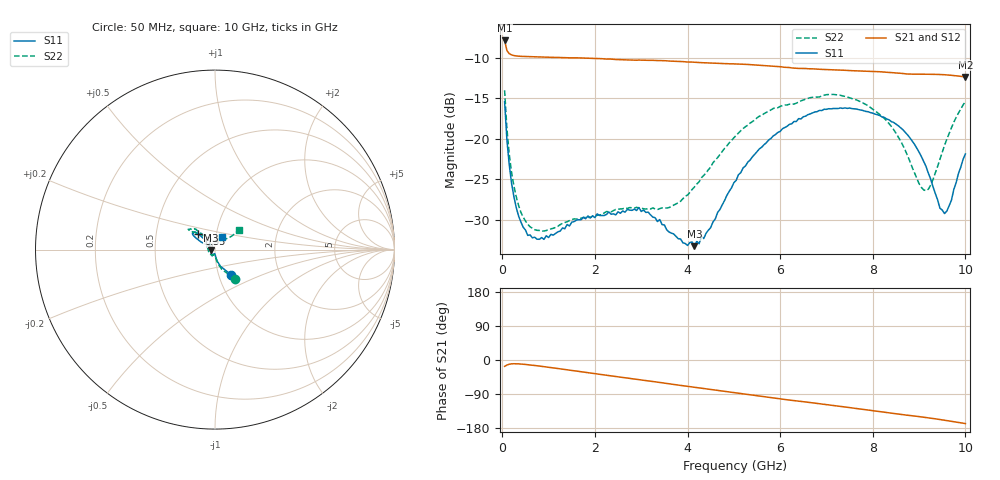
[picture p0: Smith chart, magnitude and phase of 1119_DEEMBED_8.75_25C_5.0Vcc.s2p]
!Hittite Microwave Corp.
!Digital Attenuator/PhaseShifter Rev 1.4.0
!Filename: C:\DATA\DATA\1119_DEEMBED_8.75_25C_5.0Vcc.s2p
!VNA ID: Agilent Technologies,N5224A,MY51441122,A.10.45.03
!Device type:
!2 Port Calibration.
!Temp(C): 25
!Lot Number:
!Serial Number:
!Operator:
!Misc:
!Attenuator:  8.750
# GHZ S DB R 50.0
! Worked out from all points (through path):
!   200 points, 50 MHz to 10 GHz, reference 50 ohm
!   highest |S21| = -7.89 dB at 50 MHz (marker M1); lowest = -12.4 dB at 10 GHz (marker M2)
!   group delay of S21, straight-line fit = 45 ps
!   lowest |S11| = -33.3 dB at 4.15 GHz (marker M3), VSWR 1.04, Z = 47.9 - j0.255 ohm
!   |S11| at or under -10 dB: start of sweep to end of sweep
!   |S22| runs from -31.4 to -14.0 dB; largest |S21 - S12| = 0.00082
!   S11 on the Smith chart (normalised r, x): 50 MHz: 1.15, -0.34; 6.35 GHz: 0.82, +0.15; 10 GHz: 1.07, +0.15
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0.05  -15.45 -57.1  -7.89 -16.7  -7.88 -16.7  -14.04 -55.8
0.1  -20.18 -71.9  -9.14 -13.3  -9.14 -13.3  -18.76 -71.2
0.15  -23.23 -78.0  -9.52 -11.2  -9.52 -11.2  -21.91 -77.8
0.25  -27.13 -83.4  -9.75 -9.9  -9.76 -9.9  -25.82 -83.8
0.4  -30.26 -88.2  -9.85 -10.6  -9.85 -10.6  -29.07 -87.6
0.55  -31.94 -91.1  -9.89 -12.4  -9.89 -12.4  -30.57 -90.5
0.9  -32.43 -97.9  -9.94 -17.6  -9.95 -17.6  -31.40 -96.0
1.75  -29.71 -112.8  -10.06 -31.7  -10.07 -31.7  -29.74 -109.2
2.95  -28.50 -118.0  -10.31 -51.6  -10.32 -51.6  -28.56 -146.9
3.4  -29.99 -130.4  -10.37 -59.2  -10.38 -59.3  -28.64 -167.3
4.15  -33.27 -173.0  -10.58 -72.1  -10.59 -72.1  -25.96 152.9
4.5  -30.98 159.1  -10.68 -77.7  -10.70 -77.8  -23.52 139.8
5.05  -25.16 139.0  -10.79 -86.7  -10.81 -86.7  -19.61 130.9
5.55  -21.27 135.7  -10.96 -95.2  -10.97 -95.2  -17.24 131.7
6.35  -17.89 136.6  -11.31 -107.9  -11.32 -107.9  -15.63 137.1
6.7  -16.83 138.8  -11.39 -113.1  -11.40 -113.1  -14.90 140.0
7.65  -16.35 145.3  -11.64 -127.9  -11.65 -128.0  -15.23 143.5
8.35  -17.67 148.1  -11.82 -139.4  -11.82 -139.4  -18.14 133.6
8.8  -19.89 150.2  -12.04 -146.4  -12.04 -146.4  -22.79 117.5
9.15  -23.43 150.4  -12.06 -151.7  -12.08 -151.8  -26.42 83.1
9.55  -29.25 107.3  -12.12 -159.0  -12.13 -159.0  -20.82 42.9
10  -21.90 62.4  -12.38 -167.7  -12.38 -167.7  -15.43 39.1
